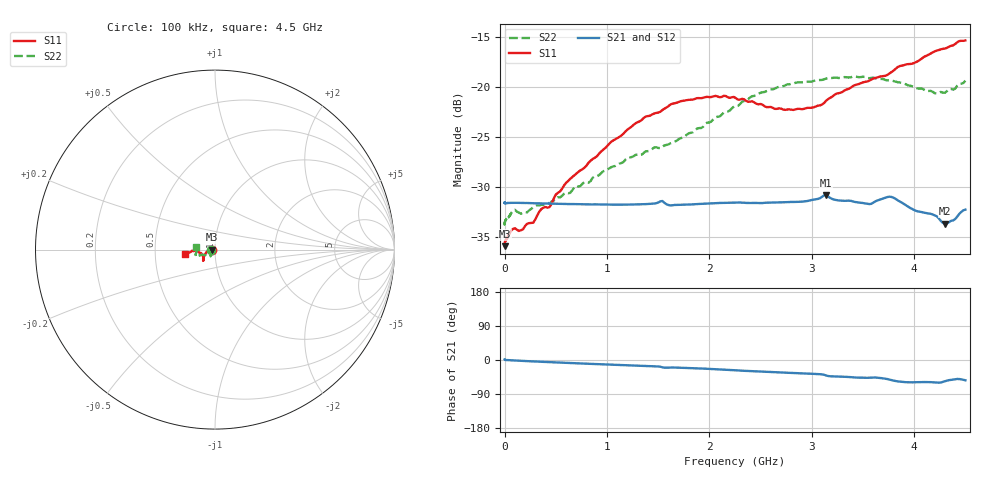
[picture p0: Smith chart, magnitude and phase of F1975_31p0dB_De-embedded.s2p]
! Integrated Device Technology
! Corporate Headquarters
! 6024 Silver Creek Valley Road
! San Jose, CA 95138  USA
! Phone:  1-408-284-8200
! Toll Free:  1-800-223-1366
! Webpage:  http://www.idt.com/
! Timing and RF Division
! 515 Groton Road, Suite 102
! Westford, MA 01886-6024
! Device:  F1975
! Description: 6-bit, 75 ohm, 0.5 dB Digital Step Attenuator
! Frequency:  5.0 MHz -  3.00 GHz
! Package:  4x4 mm QFN Plastic Package: 20 pin
! Ports:  2 RF, 11 DC
!  Pin  1  = D5 (16 dB)
!  Pin  2  = RF1  =  Port 1
!  Pin  3  = Serial Data In (DATA)
!  Pin  4  = Serial Clock (CLK)
!  Pin  5  = Serial Latch Enable (LE)
!  Pin  6  = VDD
!  Pin  7  = NC
!  Pin  8  = NC
!  Pin  9  = NC
!  Pin 10  = GND
!  Pin 11  = GND
!  Pin 12  = NC
!  Pin 13  = VMODE
!  Pin 14  = RF2  =  Port 2
!  Pin 15  = D4 (8 dB)
!  Pin 16  = D3 (4 dB)
!  Pin 17  = D2 (2 dB)
!  Pin 18  = NC
!  Pin 19  = D1 (1 dB)
!  Pin 20  = D0 (0.5 dB)
! State:  62
! Atten State:  31.0 dB
! Voltage:  +3.30 Volts
! Current:  0.592 mA
! Data:  The device was measured on a F1975 evaluation board which has
!  individual transmission lines to the RF pins.  Data was collected
!  using a calibrated network analyzer.  The evaluation board was
!  de-embedded using Automatic Fixture Removal (AFR).
!  The reference plane is the edge of the package pin.
! Misc:
!  Action Tracker AT0415
! Date Measured:  2018-02-08
! Date:  2018-03-26  MJV
! Note:
!  Integrated Device Technology supplies this data as a sample of measured
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# GHz S dB R 75
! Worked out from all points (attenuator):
!   291 points, 100 kHz to 4.5 GHz, reference 75 ohm
!   highest |S21| = -30.84 dB at 3.14 GHz (marker M1); lowest = -33.7 dB at 4.3 GHz (marker M2)
!   lowest |S11| = -35.9 dB at 100 kHz (marker M3), VSWR 1.03, Z = 72.6 - j0.00962 ohm
!   |S11| at or under -10 dB: start of sweep to end of sweep
!   |S22| runs from -33.8 to -19.0 dB; largest |S21 - S12| = 0.0002
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0.0001  -35.94 -179.8  -31.59 1.4  -31.57 1.4  -33.75 -179.0
0.007  -35.40 -178.5  -31.64 0.2  -31.63 0.1  -33.37 -177.5
0.08  -34.23 -176.1  -31.61 -1.0  -31.61 -1.0  -32.39 -169.5
0.16  -34.35 -177.4  -31.62 -2.1  -31.63 -2.1  -32.70 -160.0
0.28  -33.60 179.3  -31.65 -3.7  -31.65 -3.7  -32.04 -152.0
0.36  -32.22 179.7  -31.68 -4.7  -31.67 -4.7  -31.80 -144.6
0.44  -32.03 -179.8  -31.69 -5.6  -31.68 -5.6  -31.71 -139.1
0.5  -30.79 -180.0  -31.70 -6.4  -31.70 -6.3  -31.18 -138.1
0.76  -28.26 -169.5  -31.75 -9.3  -31.76 -9.3  -29.70 -129.1
1.28  -23.66 -153.2  -31.77 -14.8  -31.77 -14.8  -26.82 -124.8
1.52  -22.52 -145.9  -31.47 -17.6  -31.47 -17.6  -26.14 -131.3
1.64  -21.71 -143.1  -31.86 -19.8  -31.85 -19.8  -25.58 -135.3
1.88  -21.15 -139.1  -31.74 -21.9  -31.74 -21.9  -24.19 -147.2
2.26  -21.17 -137.6  -31.59 -27.2  -31.58 -27.2  -21.95 -158.0
2.64  -22.23 -147.8  -31.58 -32.1  -31.57 -32.0  -20.20 -159.5
3.02  -22.07 -164.5  -31.29 -36.6  -31.29 -36.6  -19.43 -160.3
3.14  -21.41 -167.3  -30.84 -40.9  -30.84 -40.9  -19.20 -160.7
3.56  -19.42 -177.7  -31.73 -46.7  -31.73 -46.7  -19.16 -166.2
3.76  -18.68 -176.2  -31.00 -51.8  -31.00 -51.8  -19.39 -170.0
4.22  -16.40 -173.1  -32.96 -59.5  -32.96 -59.5  -20.68 177.4
4.3  -16.20 -172.6  -33.68 -56.4  -33.67 -56.4  -20.62 177.0
4.5  -15.39 -172.0  -32.29 -53.7  -32.29 -53.7  -19.41 173.3
